FUNCTION FC 115 : VOID
TITLE =BLOCK FOR DIE_SAFETY AND DIE_CODING
AUTHOR : Esposito
FAMILY : EGAL_srl
NAME : DIE_SA_C
VERSION : 0.1

BEGIN
NETWORK
TITLE =DIE SAFETY PROXIMITY NUMBER ONE
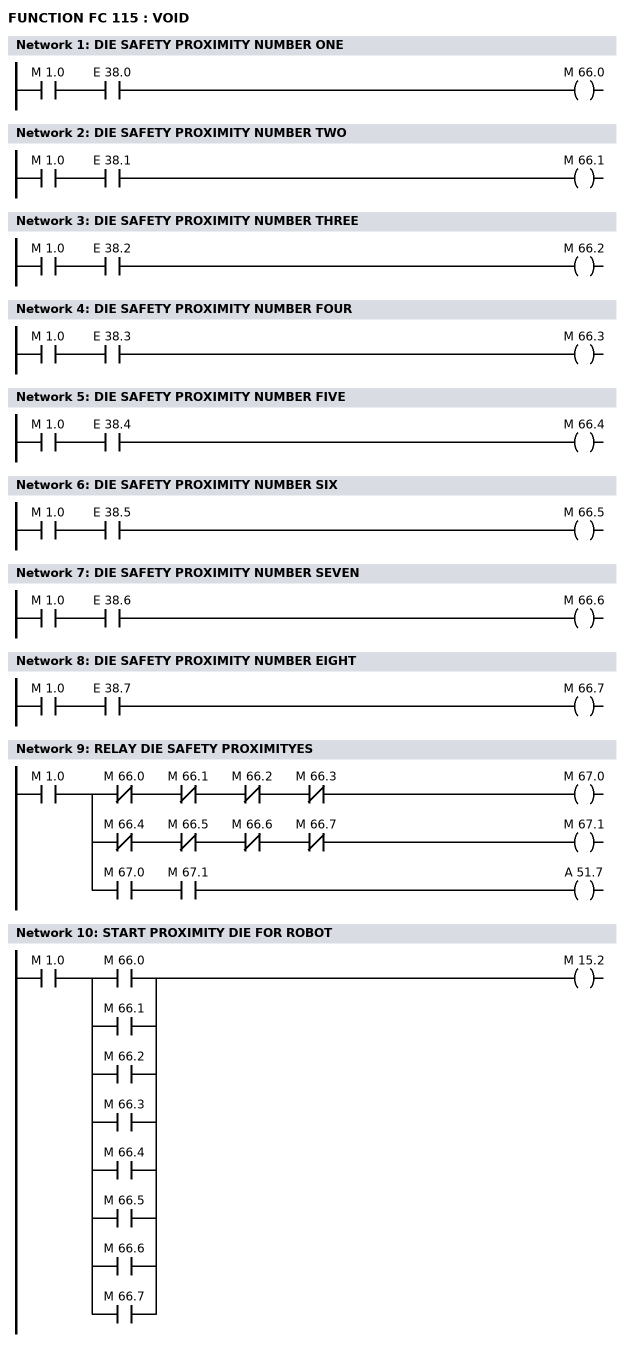
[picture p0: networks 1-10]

      U     M      1.0;
      U     E     38.0;
      =     M     66.0;
NETWORK
TITLE =DIE SAFETY PROXIMITY NUMBER TWO

      U     M      1.0;
      U     E     38.1;
      =     M     66.1;
NETWORK
TITLE =DIE SAFETY PROXIMITY NUMBER THREE

      U     M      1.0;
      U     E     38.2;
      =     M     66.2;
NETWORK
TITLE =DIE SAFETY PROXIMITY NUMBER FOUR

      U     M      1.0;
      U     E     38.3;
      =     M     66.3;
NETWORK
TITLE =DIE SAFETY PROXIMITY NUMBER FIVE

      U     M      1.0;
      U     E     38.4;
      =     M     66.4;
NETWORK
TITLE =DIE SAFETY PROXIMITY NUMBER SIX

      U     M      1.0;
      U     E     38.5;
      =     M     66.5;
NETWORK
TITLE =DIE SAFETY PROXIMITY NUMBER SEVEN

      U     M      1.0;
      U     E     38.6;
      =     M     66.6;
NETWORK
TITLE =DIE SAFETY PROXIMITY NUMBER EIGHT

      U     M      1.0;
      U     E     38.7;
      =     M     66.7;
NETWORK
TITLE =RELAY DIE SAFETY PROXIMITYES

      U     M      1.0;
      =     L      0.0;
      U     L      0.0;
      UN    M     66.0;
      UN    M     66.1;
      UN    M     66.2;
      UN    M     66.3;
      =     M     67.0;
      U     L      0.0;
      UN    M     66.4;
      UN    M     66.5;
      UN    M     66.6;
      UN    M     66.7;
      =     M     67.1;
      U     L      0.0;
      U     M     67.0;
      U     M     67.1;
      =     A     51.7;
NETWORK
TITLE =START PROXIMITY DIE FOR ROBOT

      U     M      1.0;
      U(    ;
      O     M     66.0;
      O     M     66.1;
      O     M     66.2;
      O     M     66.3;
      O     M     66.4;
      O     M     66.5;
      O     M     66.6;
      O     M     66.7;
      )     ;
      =     M     15.2;
END_FUNCTION

